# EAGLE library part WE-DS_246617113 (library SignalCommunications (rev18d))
WE-DS D-SUB-Filter Connectors Bent 90° Characteristics Standard type filtered with 1000 pF High attenuation of more than 40 dB @ 180 MHz Low size: 6.3 mm Rated voltage: 125 VDC Rated current @ 20 ºC: 5 A Withstand voltage: 250 VRMS Insulation resistance: min. 1000 MΩ Operating temperature: –55 ºC to +125 ºC Applications Filtering of interfaces External connection to -printer -sensor -display Details see: http://katalog.we-online.de/en/pbs/D-SUB-Filter Bent 90° Created on 2015-05-04 2015 (C) Wurth Elektronik
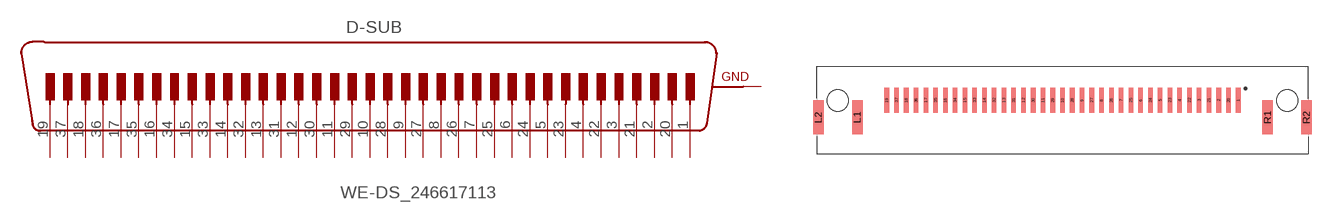
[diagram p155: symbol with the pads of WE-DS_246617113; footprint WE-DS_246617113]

Designator prefix D-SUB

## WE-DS_246617113 (WE-NUMBER: 246617113/37Pins_female)  [WE-DS_246617113]
1  19  pas
2  18  pas
3  17  pas
4  16  pas
5  15  pas
6  14  pas
7  13  pas
8  12  pas
9  11  pas
10  10  pas
11  9  pas
12  8  pas
13  7  pas
14  6  pas
15  5  pas
16  4  pas
17  3  pas
18  2  pas
19  1  pas
20  37  pas
21  36  pas
22  35  pas
23  34  pas
24  33  pas
25  32  pas
26  31  pas
27  30  pas
28  29  pas
29  28  pas
30  27  pas
31  26  pas
32  25  pas
33  24  pas
34  23  pas
35  22  pas
36  21  pas
37  20  pas
L1  GND  pwr
L2  GND  pwr
R1  GND  pwr
R2  GND  pwr

## Footprint WE-DS_246617113 (pad centres in mm)
smd 0.65 x 3.5: 1 24.84,1.38; 2 22.08,1.38; 3 19.32,1.38; 4 16.56,1.38; 5 13.8,1.38; 6 11.04,1.38; 7 8.28,1.38; 8 5.52,1.38; 9 2.76,1.38; 10 0,1.38; 11 -2.76,1.38; 12 -5.52,1.38; 13 -8.28,1.38; 14 -11.04,1.38; 15 -13.8,1.38; 16 -16.56,1.38; 17 -19.32,1.38; 18 -22.08,1.38; 19 -24.84,1.38; 20 23.46,1.38; 21 20.7,1.38; 22 17.94,1.38; 23 15.18,1.38; 24 12.42,1.38; 25 9.66,1.38; 26 6.9,1.38; 27 4.14,1.38; 28 1.38,1.38; 29 -1.38,1.38; 30 -4.14,1.38; 31 -6.9,1.38; 32 -9.66,1.38; 33 -12.42,1.38; 34 -15.18,1.38; 35 -17.94,1.38; 36 -20.7,1.38; 37 -23.46,1.38
smd 1.5 x 4.8: L1 -29,-1.05; L2 -34.5,-1.05; R1 29,-1.05; R2 34.5,-1.05
hole 3 at -31.75,1.35
hole 3 at 31.75,1.35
